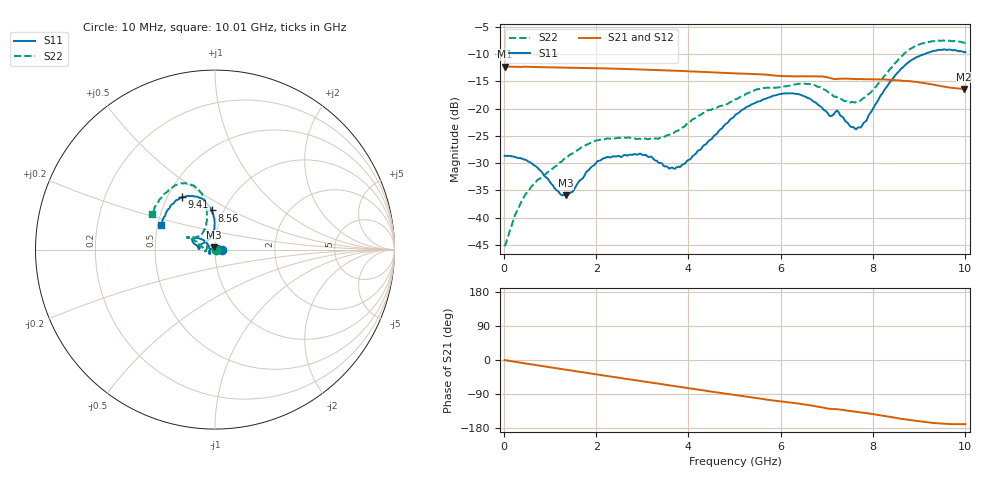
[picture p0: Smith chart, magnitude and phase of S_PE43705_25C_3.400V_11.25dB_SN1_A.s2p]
! Device ID: PE43705
! Serial: 1
! Insertion: A
! Impedance: 50 ohm
! Temp: 25C
! VDD: 3.400V
! Attenuation Step: 11.25dB
#  Hz  S  RI  R  50
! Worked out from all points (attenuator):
!   401 points, 10 MHz to 10.01 GHz, reference 50 ohm
!   highest |S21| = -12.28 dB at 10 MHz (marker M1); lowest = -16.4 dB at 9.985 GHz (marker M2)
!   lowest |S11| = -35.9 dB at 1.335 GHz (marker M3), VSWR 1.03, Z = 49.2 + j1.35 ohm
!   |S11| at or under -10 dB: start of sweep to 9.122 GHz
!   |S22| runs from -45.2 to -7.5 dB; largest |S21 - S12| = 0.002
!   S11 on the Smith chart (normalised r, x): 10 MHz: 1.08, +0.00; 8.56 GHz: 0.88, +0.40; 9.41 GHz: 0.59, +0.39; 10.01 GHz: 0.52, +0.16
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1e7  0.0369 0.000156  0.2433 -0.00106  0.2436 -0.00101  0.00546 0.00041
2.6e8  0.0346 0.0088  0.2409 -0.0218  0.2408 -0.0217  0.00475 0.00999
4.85e8  0.0295 0.016  0.2383 -0.0399  0.2384 -0.0396  0.000661 0.0168
1.335e9  -0.00816 0.0138  0.2148 -0.1022  0.2149 -0.1021  -0.0318 0.0155
1.685e9  -0.0224 0.00326  0.2004 -0.1251  0.2004 -0.1251  -0.0437 0.00721
2.21e9  -0.0326 -0.0143  0.1742 -0.1555  0.1743 -0.1554  -0.0526 -0.00616
2.96e9  -0.0311 -0.0231  0.129 -0.1888  0.129 -0.1887  -0.0522 -0.00702
3.36e9  -0.0268 -0.0172  0.1026 -0.2007  0.1029 -0.2004  -0.0532 -0.00378
3.86e9  -0.0302 0.00341  0.0685 -0.2104  0.0687 -0.2103  -0.0663 0.0098
5.01e9  -0.0673 0.0549  -0.008 -0.2105  -0.00768 -0.2107  -0.1111 0.0487
5.985e9  -0.121 0.0625  -0.0647 -0.1887  -0.0636 -0.1886  -0.1419 0.068
6.685e9  -0.1144 0.0316  -0.1004 -0.1705  -0.1004 -0.1703  -0.1503 0.0678
7.06e9  -0.0852 0.0119  -0.1195 -0.1492  -0.1195 -0.1498  -0.1201 0.0701
7.235e9  -0.094 0.017  -0.12 -0.1438  -0.1198 -0.1441  -0.1057 0.0694
7.36e9  -0.0766 0.0306  -0.1259 -0.1407  -0.1254 -0.1406  -0.0933 0.0738
7.685e9  -0.0367 0.0567  -0.1373 -0.1268  -0.137 -0.1271  -0.0684 0.0959
8.36e9  -0.00365 0.1724  -0.159 -0.0931  -0.1581 -0.0936  -0.0471 0.2218
8.56e9  -0.0181 0.2179  -0.1639 -0.0794  -0.1623 -0.0803  -0.058 0.278
8.935e9  -0.0726 0.2854  -0.1662 -0.0583  -0.1656 -0.0571  -0.1209 0.3577
9.41e9  -0.1838 0.2915  -0.1593 -0.0357  -0.1589 -0.0359  -0.2206 0.3593
9.985e9  -0.2951 0.1442  -0.1489 -0.0282  -0.1492 -0.0288  -0.3449 0.2065
1.001e10  -0.3017 0.135  -0.1493 -0.0286  -0.1499 -0.0294  -0.3531 0.1957
